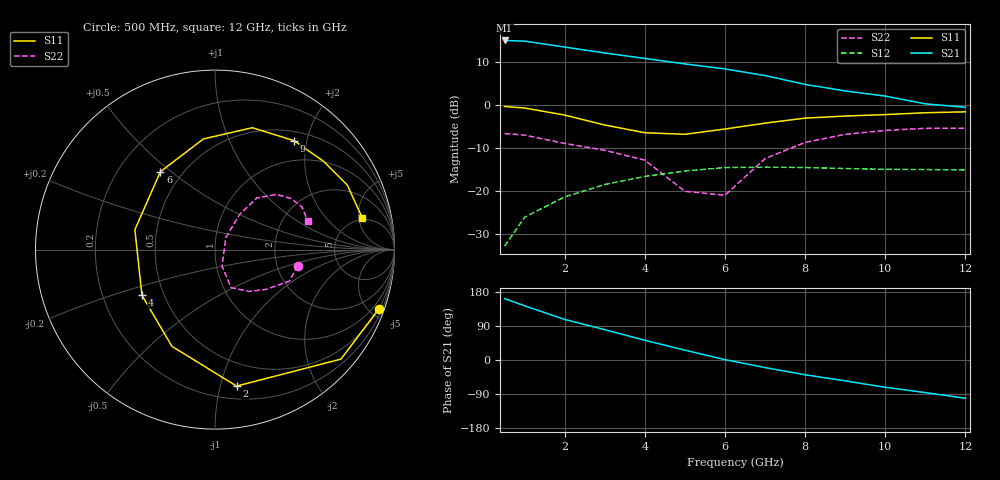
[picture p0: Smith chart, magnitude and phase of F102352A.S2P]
!ATF-10235
!S-PARAMETERS at Vds=2V  Id=25mA.  LAST UPDATED 07-22-92
# ghz s ma r 50
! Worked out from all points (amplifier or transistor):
!   13 points, 500 MHz to 12 GHz, reference 50 ohm
!   highest |S21| = 15.1 dB at 500 MHz (marker M1)
!   |S21| within 3 dB of that: start of sweep to 3.066 GHz
!   unconditionally stable (mu >= 1): 5.33 GHz to end of sweep
!   at 2 GHz: K = 0.60, MSG = 17.4 dB, |S12| = -21.3 dB
!   at 6 GHz: K = 1.01, MAG = 10.9 dB, |S12| = -14.5 dB
!   at 12 GHz: K = 1.09, MAG = 5.5 dB, |S12| = -15.0 dB
!   lowest NFmin = 0.40 dB at 500 MHz
!   S11 on the Smith chart (normalised r, x): 500 MHz: 0.50, -5.63; 2 GHz: 0.30, -1.13; 4 GHz: 0.38, -0.25; 6 GHz: 0.38, +0.46; 9 GHz: 0.64, +1.78; 12 GHz: 4.72, +5.61
0.5  0.97 -20.0  5.68 162.0  0.023 76.0  0.47 -11.0
1  0.93 -41.0  5.58 143.0  0.05 71.0  0.45 -23.0
2  0.77 -81.0  4.76 107.0  0.086 51.0  0.36 -38.0
3  0.59 -114.0  4.06 80.0  0.12 35.0  0.3 -51.0
4  0.48 -148.0  3.51 52.0  0.149 18.0  0.23 -67.0
5  0.46 166.0  3.03 26.0  0.172 3.0  0.1 -67.0
6  0.53 125.0  2.65 1.0  0.189 -14.0  0.09 48.0
7  0.62 96.0  2.22 -20.0  0.191 -28.0  0.24 55.0
8  0.71 73.0  1.75 -39.0  0.189 -41.0  0.37 51.0
9  0.75 54.0  1.47 -55.0  0.184 -46.0  0.46 42.0
10  0.78 39.0  1.28 -72.0  0.18 -59.0  0.51 34.0
11  0.82 26.0  1.04 -86.0  0.179 -71.0  0.54 26.0
12  0.84 12.0  0.95 -101.0  0.177 -82.0  0.54 17.0
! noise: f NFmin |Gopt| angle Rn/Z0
0.5  0.4  0.94  16  0.78
1  0.5  0.87  36  0.63
2  0.6  0.73  74  0.33
4  0.8  0.45  148  0.15
6  1  0.42  -137  0.12
8  1.3  0.49  -80  0.45
12  1.6  0.65  -20  1.16
